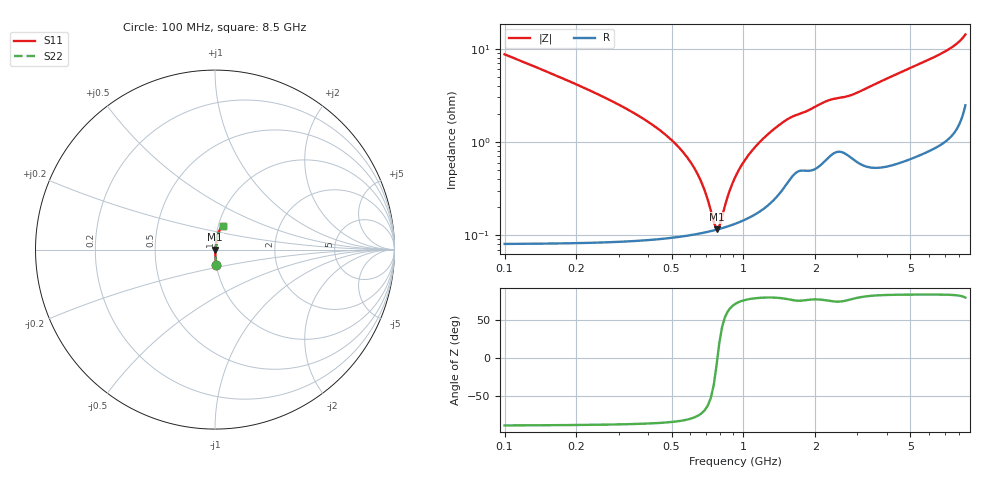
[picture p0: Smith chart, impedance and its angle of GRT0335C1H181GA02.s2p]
!Murata Part Number: GRT0335C1H181GA02
!These Parameters are Measured in Series Mode Connection
!Data Generated on Jun 19, 2026
!  o--ll--o
!Port1  Port2
!  o------o
!Operation Temp=25[degC], DC Bias Voltage=0[V]
!Freq. Start=100[MHz] Stop=9[GHz] 401[Steps]
# Hz S RI R 50
!Freq.(Hz) S11(Real) S11(Imag) S21(Real) S21(Imag) S12(Real) S12(Imag) S22(Real) S22(Imag)
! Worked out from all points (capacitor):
!   401 points, 100 MHz to 8.5 GHz, reference 50 ohm
!   read as one part in series: C = 180 pF near 142 MHz
!   lowest |Z| = 116 mohm at 772 MHz (marker M1)
!   series resonance near 778.4 MHz, so ESL is about 230 pH
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1e8  0.00829 -0.0862  0.9917 0.0862  0.9917 0.0862  0.00829 -0.0862
2.47e8  0.00186 -0.0321  0.9981 0.0321  0.9981 0.0321  0.00186 -0.0321
4.78e8  0.00105 -0.0115  0.9989 0.0115  0.9989 0.0115  0.00105 -0.0115
5.83e8  0.00103 -0.00668  0.999 0.00668  0.999 0.00668  0.00103 -0.00668
6.67e8  0.00106 -0.00354  0.9989 0.00354  0.9989 0.00354  0.00106 -0.00354
7.3e8  0.0011 -0.00147  0.9989 0.00147  0.9989 0.00147  0.0011 -0.00147
7.51e8  0.00112 -0.000817  0.9989 0.000817  0.9989 0.000817  0.00112 -0.000817
7.72e8  0.00114 -0.000186  0.9989 0.000186  0.9989 0.000186  0.00114 -0.000186
7.93e8  0.00116 0.000429  0.9988 -0.000429  0.9988 -0.000429  0.00116 0.000429
8.14e8  0.00119 0.00103  0.9988 -0.00103  0.9988 -0.00103  0.00119 0.00103
8.77e8  0.00127 0.00275  0.9987 -0.00275  0.9987 -0.00275  0.00127 0.00275
9.19e8  0.00133 0.00384  0.9987 -0.00384  0.9987 -0.00384  0.00133 0.00384
9.82e8  0.00144 0.00541  0.9986 -0.00541  0.9986 -0.00541  0.00144 0.00541
1.045e9  0.00156 0.00692  0.9984 -0.00692  0.9984 -0.00692  0.00156 0.00692
1.234e9  0.00209 0.0112  0.9979 -0.0112  0.9979 -0.0112  0.00209 0.0112
1.507e9  0.00371 0.0166  0.9963 -0.0166  0.9963 -0.0166  0.00371 0.0166
2.221e9  0.00707 0.0262  0.9929 -0.0262  0.9929 -0.0262  0.00707 0.0262
2.914e9  0.00732 0.0317  0.9927 -0.0317  0.9927 -0.0317  0.00732 0.0317
4.3e9  0.00832 0.0512  0.9917 -0.0512  0.9917 -0.0512  0.00832 0.0512
5.707e9  0.0125 0.0704  0.9875 -0.0704  0.9875 -0.0704  0.0125 0.0704
7.114e9  0.019 0.0926  0.981 -0.0926  0.981 -0.0926  0.019 0.0926
8.5e9  0.042 0.1307  0.958 -0.1307  0.958 -0.1307  0.042 0.1307
